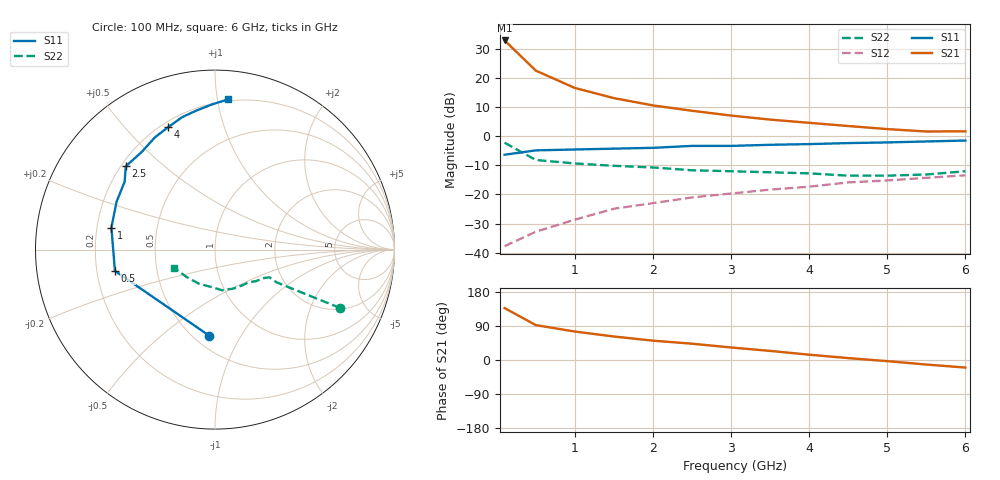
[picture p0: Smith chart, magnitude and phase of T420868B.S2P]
!AT-42086
!S-PARAMETERS at Vce=8V  Ic=35mA.  LAST UPDATED 07-21-92
# ghz s ma r 50
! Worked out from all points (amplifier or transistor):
!   13 points, 100 MHz to 6 GHz, reference 50 ohm
!   highest |S21| = 32.8 dB at 100 MHz (marker M1)
!   |S21| within 3 dB of that: start of sweep to 215.9 MHz
!   unconditionally stable (mu >= 1): 793.7 MHz to 2.411 GHz; 2.688 GHz to 3.246 GHz
!   at 1 GHz: K = 1.09, MAG = 20.8 dB, |S12| = -28.6 dB
!   at 3 GHz: K = 1.03, MAG = 12.3 dB, |S12| = -19.7 dB
!   at 6 GHz: K = 0.64, MSG = 7.5 dB, |S12| = -13.4 dB
!   S11 on the Smith chart (normalised r, x): 100 MHz: 0.59, -0.74; 500 MHz: 0.28, -0.10; 1 GHz: 0.26, +0.10; 2.5 GHz: 0.22, +0.38; 4 GHz: 0.23, +0.66; 6 GHz: 0.19, +1.07
0.1  0.48 -94.0  43.62 137.0  0.013 66.0  0.77 -25.0
0.5  0.57 -168.0  13.25 92.0  0.023 57.0  0.39 -28.0
1  0.59 168.0  6.69 75.0  0.037 62.0  0.34 -27.0
1.5  0.61 154.0  4.48 62.0  0.057 64.0  0.31 -31.0
2  0.63 143.0  3.36 51.0  0.071 61.0  0.29 -37.0
2.5  0.68 137.0  2.72 43.0  0.089 56.0  0.26 -45.0
3  0.68 127.0  2.25 33.0  0.104 58.0  0.25 -53.0
3.5  0.71 118.0  1.92 24.0  0.121 55.0  0.24 -65.0
4  0.73 111.0  1.69 14.0  0.136 49.0  0.23 -80.0
4.5  0.76 104.0  1.49 5.0  0.161 46.0  0.21 -95.0
5  0.78 98.0  1.32 -3.0  0.174 43.0  0.21 -115.0
5.5  0.81 91.0  1.2 -12.0  0.193 36.0  0.22 -136.0
6  0.84 85.0  1.208 -20.0  0.213 31.0  0.25 -156.0
